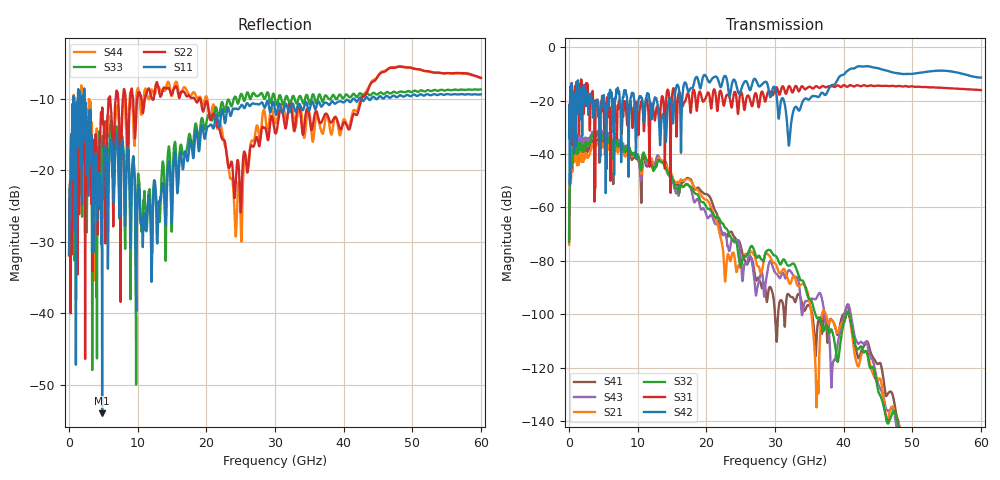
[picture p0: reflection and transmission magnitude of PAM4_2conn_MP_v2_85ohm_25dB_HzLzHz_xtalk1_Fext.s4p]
! Info: Touchstone file created by Circ.  Input file=FAB50GbE_2conn_Midplane_Examax_Topo2_v2_85ohm_25dB_HzLzHz.circ
# Hz S RI R 50
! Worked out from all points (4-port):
!   6000 points, 10 MHz to 60 GHz, reference 50 ohm
!   strongest paths, dB at 10 MHz, 15.01 GHz, 30.01 GHz, 45.01 GHz, 60 GHz:
!     S42: -34.0, -24.0, -15.3, -7.9, -11.4
!     S31: -33.9, -18.3, -15.7, -14.4, -16.1
!     S32: -72.9, -49.1, -78.0, -128.3, -168.4
!     S21: -73.9, -48.0, -81.0, -124.6, -163.7
!     S43: -71.7, -50.5, -84.4, -125.9, -172.6
!     S41: -69.4, -48.3, -100.7, -118.6, -175.3
!   lowest |S11| = -54.0 dB at 4.82 GHz (marker M1), VSWR 1.00, Z = 49.8 - j0.111 ohm
!   |S11| at or under -10 dB: start of sweep to 657 MHz; 2.263 GHz to 41.34 GHz (39.07 GHz wide, 179 % of centre); 41.56 GHz to 42.2 GHz (636.5 MHz wide, 1.52 % of centre)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
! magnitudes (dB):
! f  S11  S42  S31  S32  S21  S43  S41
! 10 MHz  -31.6  -34.0  -33.9  -72.9  -73.9  -71.7  -69.4
! 820 MHz  -14.2  -26.7  -16.9  -36.1  -39.2  -33.4  -35.7
! 4.82 GHz  -54.0  -18.8  -18.2  -33.7  -36.8  -32.2  -35.3
! 25.32 GHz  -11.0  -14.1  -19.4  -79.1  -78.8  -86.6  -78.0
! 32.06 GHz  -11.9  -36.5  -14.6  -81.9  -88.3  -83.5  -92.7
! 42.09 GHz  -10.2  -7.2  -14.3  -113.2  -119.6  -111.0  -116.1
! 60 GHz  -9.4  -11.4  -16.1  -168.4  -163.7  -172.6  -175.3
